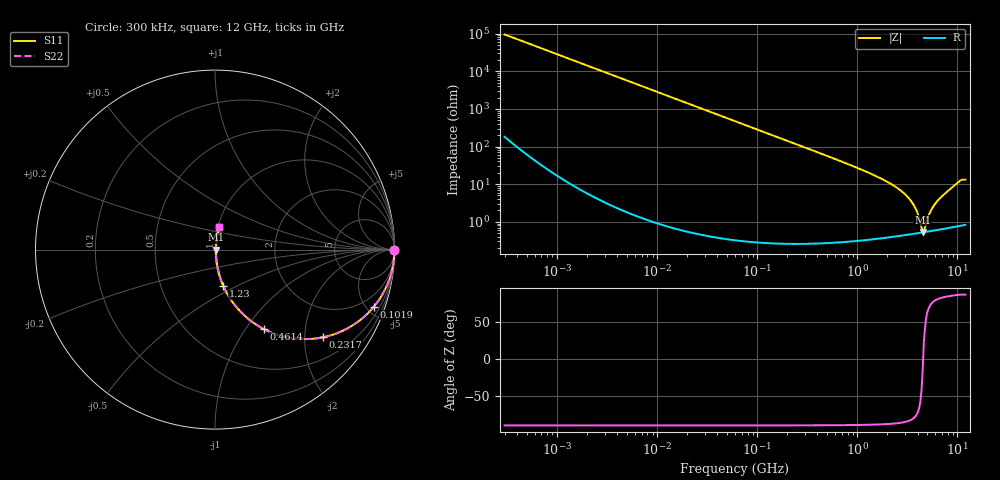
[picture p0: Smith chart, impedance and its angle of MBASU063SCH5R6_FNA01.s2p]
! MBASU063SCH5R6_FNA01  S-PARAMETER MODEL  ( Standard Model )
! Model Generated by TAIYO YUDEN Corporation (http://www.ty-top.com)
! Version 1.0
! TAIYO YUDEN Control No. 230609
! Copyright(c) 2023 TAIYO YUDEN CO.,LTD. All Rights Reserved.
! Product Description (link to TY-COMPAS)
! https://ds.yuden.co.jp/TYCOMPAS/or/detail?pn=MBASU063SCH5R6CFNA01&u=M
! Products Name : Multilayer Ceramic Capacitors
! Characteristics :
!  Capacitance : 5.6 [pF] , Rated Voltage : 50 [V] , TCC : CH / C0H
!  Case Size : 0.6 x 0.3 / 0.024 x 0.012 [mm/inch] , Thickness : 0.3 / 0.012 [mm/inch]
!  (Conditions: Temperature = 25 [degC] , DC Bias Voltage = 0 [V])
! External Node Assignments :
!  1  o---| |---o  2
! GND o---------o GND
! Frequency Range : 0.3MHz  -  12000MHz  [ 401 STEP ]
# MHZ S RI R 50
! Freq[MHz].  S11 Real  S11 Imag  S21 Real  S21 Imag  S12 Real  S12 Imag  S22 Real  S22 Imag
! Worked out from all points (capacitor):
!   401 points, 300 kHz to 12 GHz, reference 50 ohm
!   read as one part in series: C = 5.6 pF near 316.3 kHz
!   lowest |Z| = 535 mohm at 4.503 GHz (marker M1)
!   series resonance near 4.542 GHz, so ESL is about 220 pH
!   S11 on the Smith chart (normalised r, x): 300 kHz: open; 101.9 MHz: 1.01, -5.57; 231.7 MHz: 1.01, -2.45; 461.4 MHz: 1.01, -1.22; 1.23 GHz: 1.01, -0.43; 12 GHz: 1.02, +0.26
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0.3  1 -0.00106  3.13e-06 0.00106  3.13e-06 0.00106  1 -0.00106
1.769972  1 -0.00623  4.14e-05 0.00623  4.14e-05 0.00623  1 -0.00623
10.44266  0.9986 -0.0367  0.00136 0.0367  0.00136 0.0367  0.9986 -0.0367
60  0.9572 -0.2022  0.0428 0.2022  0.0428 0.2022  0.9572 -0.2022
101.9188  0.8856 -0.3178  0.1144 0.3178  0.1144 0.3178  0.8856 -0.3178
231.6935  0.5991 -0.489  0.4009 0.489  0.4009 0.489  0.5991 -0.489
353.9943  0.3892 -0.4859  0.6108 0.4859  0.6108 0.4859  0.3892 -0.4859
461.3684  0.2717 -0.4426  0.7283 0.4426  0.7283 0.4426  0.2717 -0.4426
723.8279  0.1295 -0.332  0.8705 0.332  0.8705 0.332  0.1295 -0.332
1229.528  0.0467 -0.2035  0.9533 0.2035  0.9533 0.2035  0.0467 -0.2035
2088.533  0.0151 -0.1053  0.9849 0.1053  0.9849 0.1053  0.0151 -0.1053
2795.104  0.00822 -0.0624  0.9918 0.0624  0.9918 0.0624  0.00822 -0.0624
3454.93  0.00585 -0.0344  0.9942 0.0344  0.9942 0.0344  0.00585 -0.0344
3841.137  0.00531 -0.021  0.9947 0.021  0.9947 0.021  0.00531 -0.021
4385.161  0.00516 -0.00445  0.9948 0.00445  0.9948 0.00445  0.00516 -0.00445
4502.883  0.0052 -0.00113  0.9948 0.00113  0.9948 0.00113  0.0052 -0.00113
4747.894  0.00534 0.00478  0.9947 -0.00478  0.9947 -0.00478  0.00534 0.00478
5140.631  0.00569 0.0132  0.9943 -0.0132  0.9943 -0.0132  0.00569 0.0132
5565.855  0.00617 0.0215  0.9938 -0.0215  0.9938 -0.0215  0.00617 0.0215
6354.153  0.00734 0.0357  0.9927 -0.0357  0.9927 -0.0357  0.00734 0.0357
10236.47  0.0199 0.1098  0.9801 -0.1098  0.9801 -0.1098  0.0199 0.1098
12000  0.0246 0.1266  0.9754 -0.1266  0.9754 -0.1266  0.0246 0.1266
